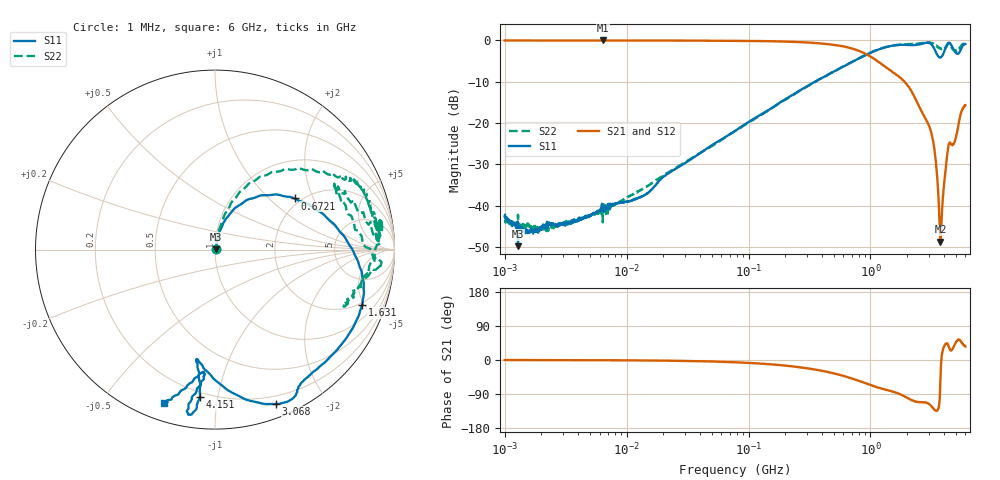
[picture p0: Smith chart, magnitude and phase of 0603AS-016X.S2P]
!s-Parameter Generated by FASTRON Sdn. Bhd.
!FASTRON P/N : 0603AS-016X
!Keysight Technologies: E5071C_MY46733604_B.14.02
!Date: Thu Nov 23 10:14:47 2023
!Version  :Rev01  Thu Nov 23 10:14:47 2023
!Data & Calibration Information:
!Freq  S11:SOLT2(ON)  S21:SOLT2(ON)  S12:SOLT2(ON)  S22:SOLT2(ON)
!PortZ  Port1:50+j0  Port2:50+j0
!When reading reference impedance value at option line is always used.
! Remarks : This data is being provided solely for informational purposes.
# Hz S dB R 50
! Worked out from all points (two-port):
!   1601 points, 1 MHz to 6 GHz, reference 50 ohm
!   highest |S21| = -0.04 dB at 6.378 MHz (marker M1); lowest = -48.7 dB at 3.746 GHz (marker M2)
!   |S21| within 3 dB of the highest: start of sweep to 877.4 MHz
!   lowest |S11| = -49.8 dB at 1.288 MHz (marker M3), VSWR 1.01, Z = 50.3 + j0.085 ohm
!   |S11| at or under -10 dB: start of sweep to 351.7 MHz
!   |S22| runs from -46.1 to -0.5 dB; largest |S21 - S12| = 0.0092
!   S11 on the Smith chart (normalised r, x): 1 MHz: 1.01, +0.01; 672.1 MHz: 1.85, +1.46; 1.631 GHz: 1.84, -4.85; 3.068 GHz: 0.12, -1.46; 4.151 GHz: 0.17, -0.89; 6 GHz: 0.08, -0.72
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1000000  -42.56 19.7  -0.05 -0.0  -0.05 -0.1  -43.34 20.4
1287650  -49.77 15.1  -0.05 -0.1  -0.05 -0.1  -42.17 8.3
4277066  -43.35 47.1  -0.06 -0.4  -0.05 -0.4  -43.27 47.6
6378092  -41.04 62.1  -0.04 -0.6  -0.08 -0.7  -44.01 60.2
1.366685e7  -37.64 73.0  -0.05 -1.1  -0.06 -1.2  -35.84 63.3
1.823719e7  -34.21 72.7  -0.06 -1.5  -0.07 -1.5  -33.44 70.1
7.757876e7  -21.89 76.8  -0.12 -6.0  -0.12 -6.0  -21.97 78.2
3.307917e8  -10.48 59.5  -0.59 -23.8  -0.59 -23.7  -10.58 69.4
6.721474e8  -5.57 32.7  -1.82 -46.6  -1.81 -46.6  -5.52 54.1
9.321099e8  -3.44 12.8  -3.42 -62.7  -3.42 -62.7  -3.36 40.7
1.414819e9  -1.46 -11.9  -7.04 -80.8  -7.05 -80.8  -1.48 26.9
1.630775e9  -1.15 -20.5  -8.37 -86.5  -8.38 -86.5  -1.11 25.0
2.27946e9  -1.15 -52.7  -13.52 -108.9  -13.51 -108.7  -0.89 9.9
3.068351e9  -0.68 -68.6  -21.25 -118.0  -21.22 -118.0  -0.59 7.1
3.381472e9  -2.42 -87.1  -27.54 -132.1  -27.53 -132.3  -1.00 -2.9
3.644712e9  -4.04 -98.4  -40.67 -121.2  -40.67 -121.2  -1.77 -19.2
3.745958e9  -4.12 -99.5  -48.72 -51.9  -48.74 -52.0  -1.95 -22.5
3.867453e9  -3.80 -98.6  -40.76 18.1  -40.77 18.2  -2.02 -22.5
4.150942e9  -1.65 -95.8  -30.53 43.6  -30.54 43.5  -1.58 -13.5
4.377169e9  -0.62 -98.7  -25.17 35.6  -25.19 35.6  -0.67 -5.0
5.048685e9  -3.14 -94.6  -23.05 48.9  -23.07 49.0  -2.47 28.4
6e9  -0.89 -108.4  -15.70 35.4  -15.70 35.6  -0.72 7.8
